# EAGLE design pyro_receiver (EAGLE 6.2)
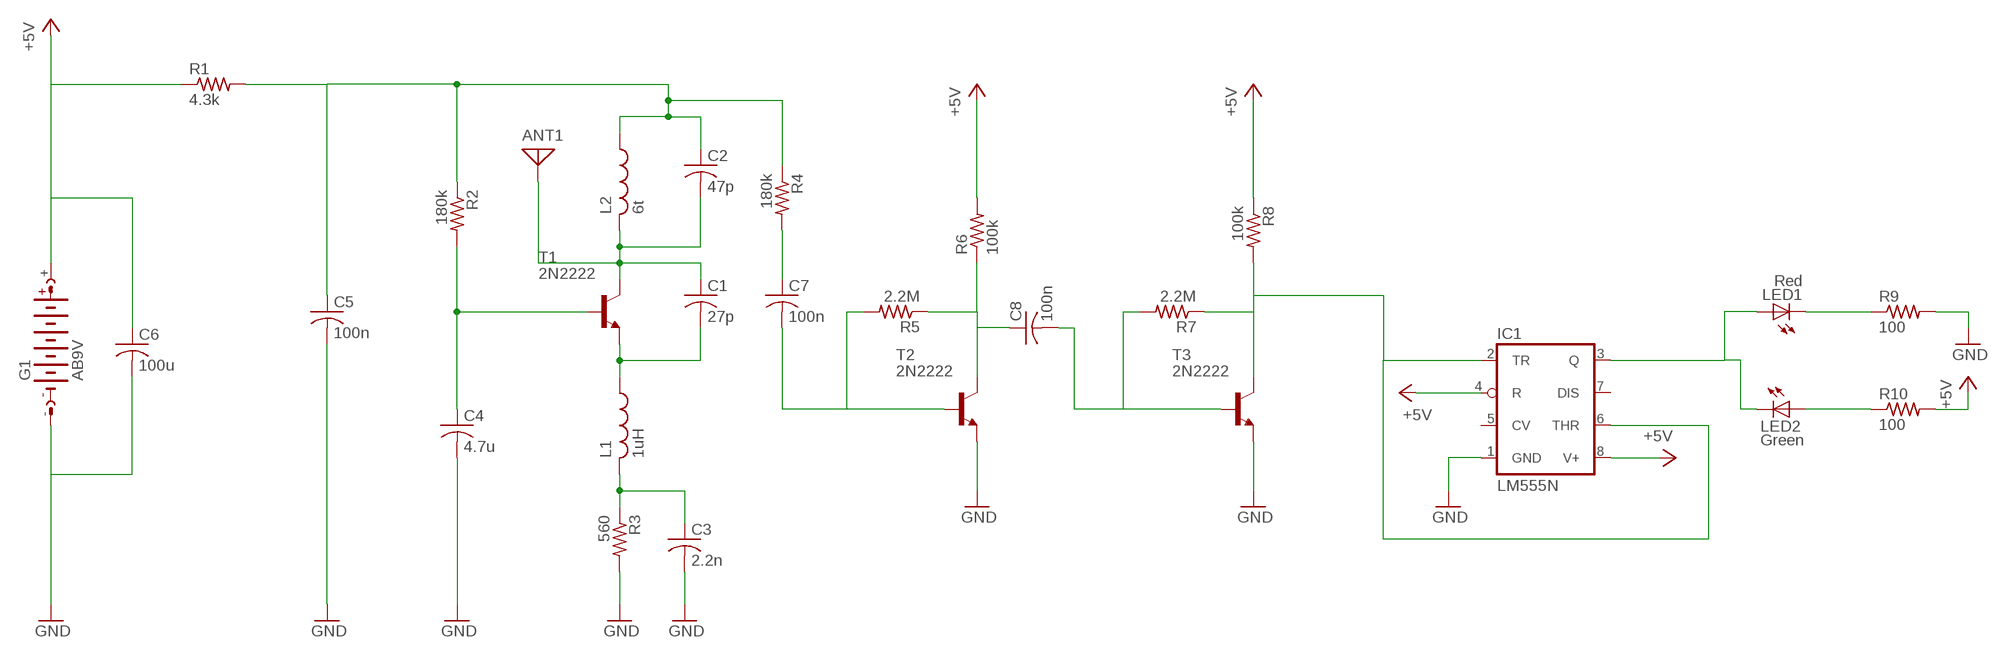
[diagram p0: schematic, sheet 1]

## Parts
ANT1  ANTENNA  [PAD-01]
C1  27p  C-US025-025X050  [C025-025X050]
C2  47p  C-US025-025X050  [C025-025X050]
C3  2.2n  C-US025-025X050  [C025-025X050]
C4  4.7u  C-US025-025X050  [C025-025X050]
C5  100n  C-US025-025X050  [C025-025X050]
C6  100u  C-US025-025X050  [C025-025X050]
C7  100n  C-US025-025X050  [C025-025X050]
C8  100n  C-US025-025X050  [C025-025X050]
G1  AB9V  [AB9V]
IC1  LM555N  [DIL08]
L1  1uH  L-US0207/12  [0207/12]
L2  6t  L-US0207/10  [0207/10]
LED1  Red  LED5MM  [LED5MM]
LED2  Green  LED5MM  [LED5MM]
R1  4.3k  R-US_0207/10  [0207/10]
R2  180k  R-US_0207/10  [0207/10]
R3  560  R-US_0207/10  [0207/10]
R4  180k  R-US_0207/10  [0207/10]
R5  2.2M  R-US_0207/10  [0207/10]
R6  100k  R-US_0207/10  [0207/10]
R7  2.2M  R-US_0207/10  [0207/10]
R8  100k  R-US_0207/10  [0207/10]
R9  100  R-US_0207/10  [0207/10]
R10  100  R-US_0207/10  [0207/10]
T1  2N2222  2N2222-NPN-TO92-EBC  [TO92-EBC]
T2  2N2222  2N2222-NPN-TO92-EBC  [TO92-EBC]
T3  2N2222  2N2222-NPN-TO92-EBC  [TO92-EBC]

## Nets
+5V: C6.1 G1.+ IC1.4(R) IC1.8(V+) R1.1 R6.2 R8.1 R10.2
GND: C3.2 C4.2 C5.2 C6.2 G1.- IC1.1(GND) R3.2 R9.2 T2.E T3.E
N$1: C8.1 R5.1 R6.1 T2.C
N$2: C2.1 C5.1 L2.1 R1.2 R2.1 R4.1
N$3: ANT1.1 C1.1 C2.2 L2.2 T1.C
N$4: C1.2 L1.1 T1.E
N$5: C4.1 R2.2 T1.B
N$6: IC1.2(TR) IC1.6(THR) R7.1 R8.2 T3.C
N$7: C8.2 R7.2 T3.B
N$8: C7.1 R4.2
N$9: C3.1 L1.2 R3.1
N$11: C7.2 R5.2 T2.B
N$12: IC1.3(Q) LED1.A LED2.K(C)
N$15: LED1.K(C) R9.1
N$16: LED2.A R10.1
Unconnected: IC1.5(CV) IC1.7(DIS)

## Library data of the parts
ANT1 = discrete:ANTENNA: Antenna
C1-C8 = resistor:C-US: CAPACITOR, American symbol
G1 = battery:AB9V: 9-V BATTERY CLIP
IC1 = linear:*555: TIMER
L1 L2 = resistor:L-US: INDUCTOR, American symbol
LED1 LED2 = led:LED: LED
R1-R10 = resistor:R-US_: RESISTOR, American symbol
T1-T3 = transistor-neu-to92:*-NPN-: NPN Transistror

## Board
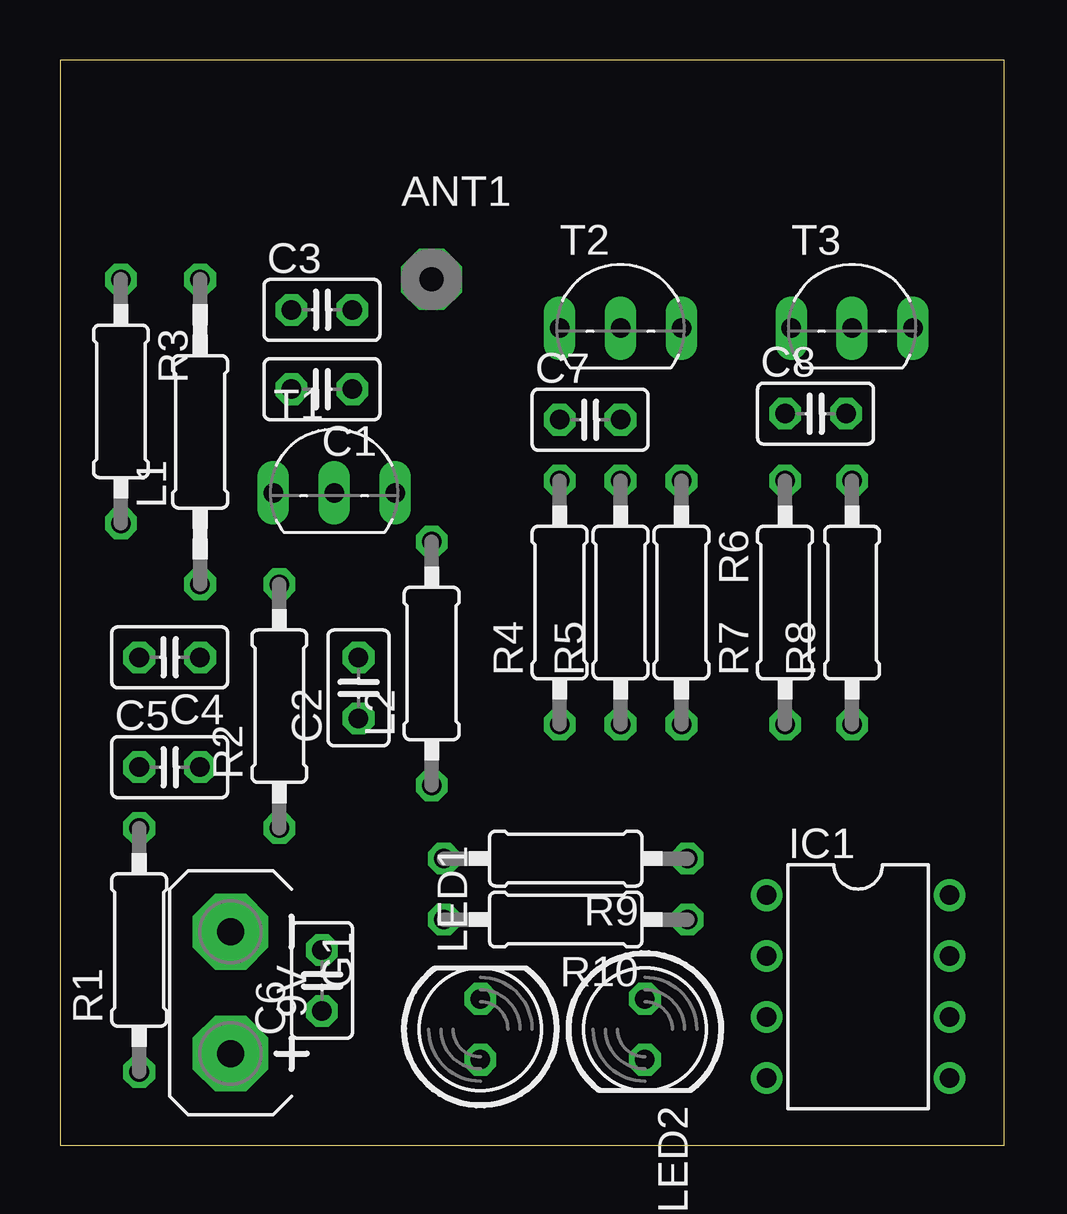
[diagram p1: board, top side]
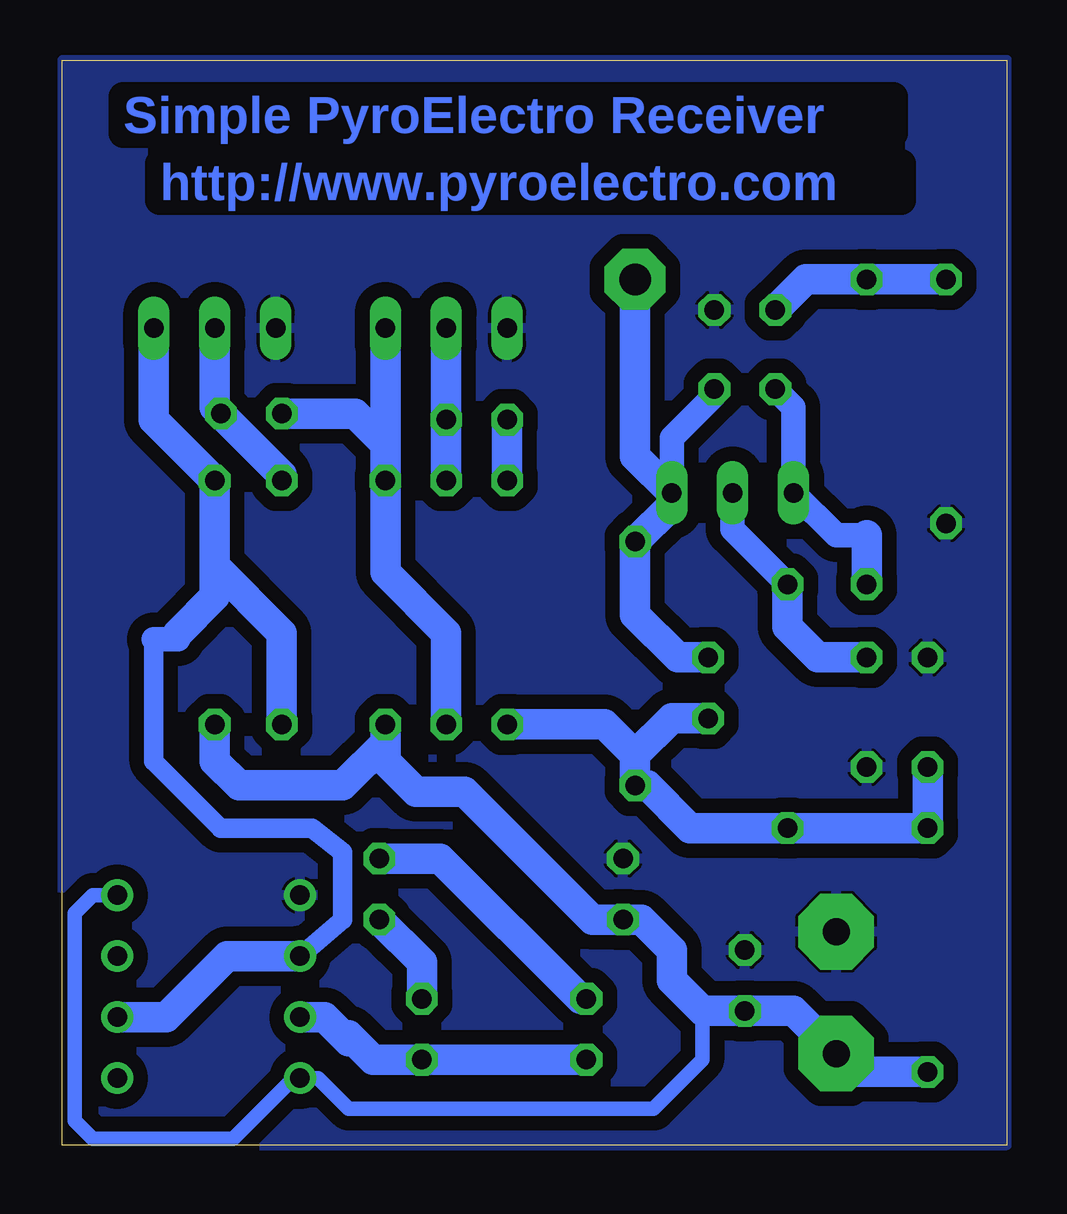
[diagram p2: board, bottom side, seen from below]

Size 39.37 x 45.21 mm. Coordinates in mm from the lower left corner, seen from the top.
Outline: 0,0 39.37,0 39.37,45.21 0,45.21 0,0
Copper layers (1*16): Top 0.035mm / dielectric 1.5mm / Bottom 0.035mm
Design rules: minimum track width 10mil, minimum drill 24mil, track to track 8mil, track to pad 8mil, pad to pad 8mil, via to via 8mil, smd to smd 8mil, copper to edge 0mil, drill to drill 8mil, minimum pad ring 10mil, minimum via ring 8mil, stop-mask expansion 4mil, vias tented up to drill 0mil, thermal gap 5mil

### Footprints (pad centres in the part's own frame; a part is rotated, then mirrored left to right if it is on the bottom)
PAD-01 = drill 1.321 pad 2.54 octagon: 1 0,0
C025-025X050 = drill 0.813 octagon: 1 -1.27,0; 2 1.27,0
AB9V = drill 1.118 pad 3.15 octagon: + 0,2.54; - 0,-2.54
DIL08 = drill 0.813 pad 1.27: 1 -3.81,-3.81; 2 -1.27,-3.81; 3 1.27,-3.81; 4 3.81,-3.81; 5 3.81,3.81; 6 1.27,3.81; 7 -1.27,3.81; 8 -3.81,3.81
0207/12 = drill 0.813 octagon: 1 -6.35,0; 2 6.35,0
0207/10 = drill 0.813 octagon: 1 -5.08,0; 2 5.08,0
LED5MM = drill 0.813 octagon: A -1.27,0; K 1.27,0
TO92-EBC = drill 0.813 long: B 0,-1.27; C 2.54,-1.27; E -2.54,-1.27

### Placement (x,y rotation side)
ANT1  15.49,36.07 0 top
C1  10.92,31.5 180 top
C2  12.45,19.05 90 top
C3  10.92,34.8 0 top
C4  4.57,20.32 180 top
C5  4.57,15.75 0 top
C6  10.92,6.86 90 top
C7  22.1,30.23 0 top
C8  31.5,30.48 0 top
G1  7.11,6.35 180 top
IC1  33.27,6.6 270 top
L1  5.84,29.72 90 top
L2  15.49,20.07 90 top
LED1  17.53,4.83 90 top
LED2  24.38,4.83 270 top
R1  3.3,8.13 90 top
R2  9.14,18.29 90 top
R3  2.54,30.99 270 top
R4  20.83,22.61 90 top
R5  23.37,22.61 90 top
R6  25.91,22.61 270 top
R7  30.23,22.61 90 top
R8  33.02,22.61 90 top
R9  21.08,11.94 180 top
R10  21.08,9.4 180 top
T1  11.43,28.45 0 top
T2  23.37,35.31 0 top
T3  33.02,35.31 0 top

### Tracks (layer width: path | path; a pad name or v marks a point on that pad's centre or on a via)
+5V
  Bottom 0.61: 12.7,5.59 12.7,3.56 14.73,1.52 27.43,1.52 28.7,2.79 IC1.4 29.72,2.54 29.97,2.54 32.26,0.25 38.1,0.25 38.86,1.02 38.86,9.65 38.1,10.41 IC1.8
  Bottom 1.27: R1.1 6.35,3.05 G1.+ 8.89,5.59 C6.1 12.7,5.59 13.97,6.86 13.97,8.13 15.24,9.4 R10.2 17.27,9.4 22.61,14.73 24.64,14.73 25.91,16 R6.2 25.91,16.76 27.69,14.99 32,14.99 33.02,16 R8.1
GND
  pour Bottom (isolate 0.61): 0,0 0,45.21 39.37,45.21 39.37,0
N$1
  Bottom 1.27: R6.1 T2.C | R5.1 23.37,21.34 25.91,23.88 R6.1 | R6.1 25.91,29.21 27.18,30.48 C8.1
N$2
  Bottom 1.27: C2.1 13.97,17.78 15.49,16.26 | 15.49,16.26 L2.1 14.99,14.99 13.21,13.21 R2.1 R1.2 C5.1 | R4.1 16.76,17.53 15.49,16.26
N$3
  Bottom 1.016: 13.97,27.94 T1.C 13.97,29.46 12.19,31.24 C1.1
  Bottom 1.27: C2.2 13.72,20.32 15.49,22.1 L2.2 13.97,26.67 T1.C 15.49,28.7 ANT1.1
N$4
  Bottom 1.016: C1.2 8.89,30.73 T1.E 7.11,25.4 5.84,25.4
  Bottom 1.27: L1.1 5.84,25.4
N$5
  Bottom 1.016: R2.2 11.43,25.65 T1.B
  Bottom 1.27: C4.1 7.87,20.32 9.14,21.59 R2.2
N$6
  Bottom 0.813: IC1.2 27.69,9.4 27.69,12.19 28.96,13.21 32.77,13.21 35.56,16 35.56,21.08
  Bottom 1.016: 35.56,21.08 34.54,21.08 34.54,21.34
  Bottom 1.27: R7.1 30.23,21.34 33.02,24.13 | 33.02,24.13 R8.2 35.56,30.23 T3.C | 33.02,24.13 33.02,22.86 34.54,21.34 | IC1.2 32.51,7.87 35.05,5.33 IC1.6
N$7
  Bottom 1.27: R7.2 30.23,27.94 C8.2 33.02,30.73 T3.B
N$8
  Bottom 1.27: R4.2 C7.1
N$9
  Bottom 1.27: C3.1 8.38,36.07 L1.2 R3.1
N$11
  Bottom 1.27: R5.2 C7.2 T2.B
N$12
  Bottom 1.27: LED1.A LED2.K 26.42,3.56 27.43,4.57 27.43,4.32 28.45,5.33 IC1.3
N$15
  Bottom 1.27: LED1.K 17.78,6.1 23.62,11.94 R9.1
N$16
  Bottom 1.27: LED2.A 24.38,7.62 R10.1

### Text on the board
Bottom: Simple PyroElectro Receiver | http://www.pyroelectro.com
